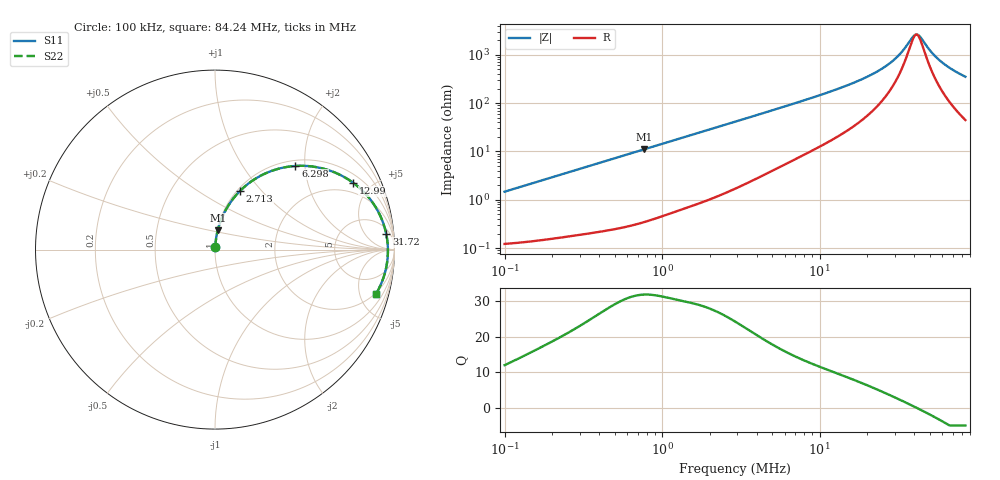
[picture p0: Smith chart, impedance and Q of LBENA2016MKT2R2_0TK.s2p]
! LBENA2016MKT2R2_0TK  S-PARAMETER MODEL  ( Standard Model )
! Model Generated by TAIYO YUDEN Corporation (http://www.ty-top.com)
! Version 1.0
! TAIYO YUDEN Control No. 20240828
! Copyright(c) 2024 TAIYO YUDEN CO.,LTD. All Rights Reserved.
! Product Description (link to TY-COMPAS)
! https://ds.yuden.co.jp/TYCOMPAS/or/detail?pn=LBENA2016MKT2R2M0TK&u=M
! Products Name : Inductors
! Characteristics :
!  Inductance : 2.2 [uH] , SRF(min) : - [Hz] , DC Resistance(max) : 0.12 [Ohm]
!  Rated Current : Saturation  2200 [mA] , Temp Rise  1800 [mA] (40 [degC])
!  Case Size : 2.0 x 1.6 / 0.079 x 0.063 [mm/inch] , Thickness : 1.2 / 0.047 [mm/inch]
!  (Conditions: Temperature = 25 [degC] , DC Bias Current = 0 [A])
! External Node Assignments :
!  1  o---GGG---o  2
! GND o---------o GND
! Frequency Range : 0.1MHz  -  84.23641MHz  [ 402 STEP ]
# MHz S RI R 50
! Freq[MHz].  S11 Real  S11 Imag  S21 Real  S21 Imag  S12 Real  S12 Imag  S22 Real  S22 Imag
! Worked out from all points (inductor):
!   401 points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, 100 kHz to 84.24 MHz, reference 50 ohm
!   read as one part in series: L = 2.33 uH near 103.4 kHz
!   highest Q = 31.9 at 767.3 kHz (marker M1), where L = 2.28 uH
!   self-resonance near 41.18 MHz
!   S11 on the Smith chart (normalised r, x): 100 kHz: 1.00, +0.03; 2.713 MHz: 1.03, +0.77; 6.298 MHz: 1.12, +1.79; 12.99 MHz: 1.40, +3.89; 31.72 MHz: 8, +18; 84.24 MHz: 1.89, -6.96
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0.1  0.00143 0.0146  0.9986 -0.0146  0.9986 -0.0146  0.00143 0.0146
0.309045  0.00388 0.0444  0.9961 -0.0444  0.9961 -0.0444  0.00388 0.0444
0.767297  0.0152 0.1078  0.9848 -0.1078  0.9848 -0.1078  0.0152 0.1078
0.955086  0.0224 0.1328  0.9776 -0.1328  0.9776 -0.1328  0.0224 0.1328
1.721962  0.0633 0.2269  0.9367 -0.2269  0.9367 -0.2269  0.0633 0.2269
2.713282  0.1382 0.3257  0.8618 -0.3257  0.8618 -0.3257  0.1382 0.3257
2.902351  0.1543 0.3413  0.8457 -0.3413  0.8457 -0.3413  0.1543 0.3413
4.2039  0.2715 0.4202  0.7285 -0.4202  0.7285 -0.4202  0.2715 0.4202
6.297706  0.4479 0.466  0.5521 -0.466  0.5521 -0.466  0.4479 0.466
8.96956  0.6164 0.4476  0.3836 -0.4476  0.3836 -0.4476  0.6164 0.4476
12.99193  0.7701 0.372  0.2299 -0.372  0.2299 -0.372  0.7701 0.372
20.12941  0.8932 0.2396  0.1068 -0.2396  0.1068 -0.2396  0.8932 0.2396
27.71995  0.9422 0.1329  0.0578 -0.1329  0.0578 -0.1329  0.9422 0.1329
31.71775  0.9539 0.0877  0.0461 -0.0877  0.0461 -0.0877  0.9539 0.0877
38.82106  0.9627 0.0199  0.0373 -0.0199  0.0373 -0.0199  0.9627 0.0199
40.15086  0.9632 0.00853  0.0368 -0.00853  0.0368 -0.00853  0.9632 0.00853
41.52622  0.9634 -0.0028  0.0366 0.0028  0.0366 0.0028  0.9634 -0.0028
43.67809  0.9632 -0.0198  0.0368 0.0198  0.0368 0.0198  0.9632 -0.0198
50.82617  0.9589 -0.0711  0.0411 0.0711  0.0411 0.0711  0.9589 -0.0711
58.15638  0.9501 -0.1171  0.0499 0.1171  0.0499 0.1171  0.9501 -0.1171
69.99203  0.9296 -0.181  0.0704 0.181  0.0704 0.181  0.9296 -0.181
84.23641  0.8981 -0.2451  0.1019 0.2451  0.1019 0.2451  0.8981 -0.2451
